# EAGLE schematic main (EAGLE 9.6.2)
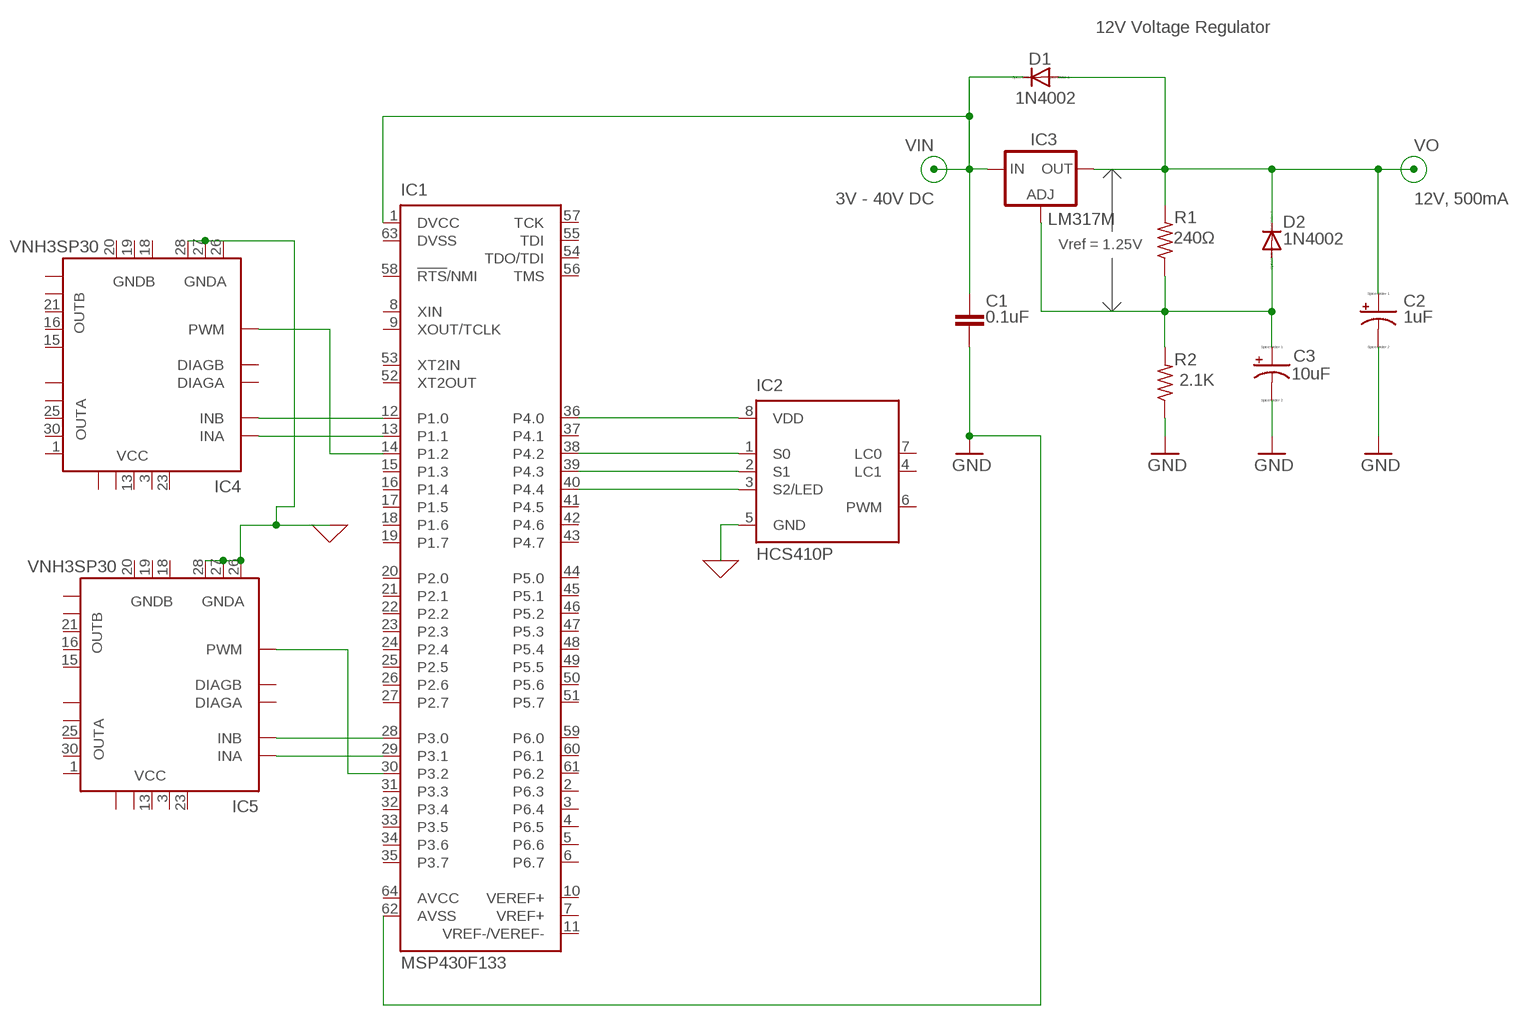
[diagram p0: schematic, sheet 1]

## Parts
C1  0.1uF  C-EU075-052X106  [C075-052X106]
C2  1uF  CPOL-US085CS-1AR  [085CS_1AR]
C3  10uF  CPOL-US085CS-1AR  [085CS_1AR]
D1  1N4002  1N4004  [DO41-10]
D2  1N4002  1N4004  [DO41-10]
IC1  MSP430F133  [SQFP-S-10X10-64]
IC2  HCS410P  [DIL8]
IC3  LM317MBSTT3  [SOT223]
IC4  VNH3SP30  [MULTIPOWERSO-30]
IC5  VNH3SP30  [MULTIPOWERSO-30]
R1  240Ω  R-US_M0805  [M0805]
R2  2.1K  R-US_M0805  [M0805]

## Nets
0: IC2.5(GND) IC4.26(GNDA) IC4.27(GNDA) IC4.28(GNDA) IC5.26(GNDA) IC5.27(GNDA) IC5.28(GNDA) ; supply symbol labelled GND
GND: C1.2 C2.- C3.- IC1.62(AVSS) R2.1
N$1: IC1.36(P4.0) IC2.8(VDD)
N$2: C3.+ D2.A IC3.1(ADJ) R1.1 R2.2
N$3: IC1.38(P4.2) IC2.1(S0)
N$4: IC1.39(P4.3) IC2.2(S1)
N$5: IC1.40(P4.4) IC2.3(S2/LED)
N$6: IC1.28(P3.0) IC5.11(INB)
N$7: IC1.29(P3.1) IC5.5(INA)
N$8: IC1.30(P3.2) IC5.8(PWM)
N$9: IC1.12(P1.0) IC4.11(INB)
N$10: IC1.13(P1.1) IC4.5(INA)
N$11: IC1.14(P1.2) IC4.8(PWM)
VIN: C1.1 D1.C IC1.1(DVCC) IC3.3(IN)
VO: C2.+ D1.A D2.C IC3.4(OUT) R1.2
Unconnected: IC1.2(P6.3) IC1.3(P6.4) IC1.4(P6.5) IC1.5(P6.6) IC1.6(P6.7) IC1.7(VREF+) IC1.8(XIN) IC1.9(XOUT/TCLK) IC1.10(VEREF+) IC1.11(VREF-/VEREF-) IC1.15(P1.3) IC1.16(P1.4) IC1.17(P1.5) IC1.18(P1.6) IC1.19(P1.7) IC1.20(P2.0) IC1.21(P2.1) IC1.22(P2.2) IC1.23(P2.3) IC1.24(P2.4) IC1.25(P2.5) IC1.26(P2.6) IC1.27(P2.7) IC1.31(P3.3) IC1.32(P3.4) IC1.33(P3.5) IC1.34(P3.6) IC1.35(P3.7) IC1.37(P4.1) IC1.41(P4.5) IC1.42(P4.6) IC1.43(P4.7) IC1.44(P5.0) IC1.45(P5.1) IC1.46(P5.2) IC1.47(P5.3) IC1.48(P5.4) IC1.49(P5.5) IC1.50(P5.6) IC1.51(P5.7) IC1.52(XT2OUT) IC1.53(XT2IN) IC1.54(TDO/TDI) IC1.55(TDI) IC1.56(TMS) IC1.57(TCK) IC1.58(!RTS!/NMI) IC1.59(P6.0) IC1.60(P6.1) IC1.61(P6.2) IC2.4(LC1) IC2.6(PWM) IC2.7(LC0) IC4.1(OUTA) IC4.6(DIAGA) IC4.10(DIAGB) IC4.15(OUTB) IC4.16(OUTB) IC4.21(OUTB) IC4.25(OUTA) IC4.30(OUTA) IC4.OUTA IC4.OUTA@1(OUTA) IC4.OUTB IC4.OUTB@1(OUTB) IC5.1(OUTA) IC5.6(DIAGA) IC5.10(DIAGB) IC5.15(OUTB) IC5.16(OUTB) IC5.21(OUTB) IC5.25(OUTA) IC5.30(OUTA) IC5.OUTA IC5.OUTA@1(OUTA) IC5.OUTB IC5.OUTB@1(OUTB)

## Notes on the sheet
- 12V Voltage Regulator
- 3V - 40V DC | 12V, 500mA
- Vref = 1.25V

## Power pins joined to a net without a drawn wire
AVCC: IC1.64(AVCC)
DVSS: IC1.63(DVSS)
GNDB: IC4.18(GNDB) IC4.19(GNDB) IC4.20(GNDB) IC5.18(GNDB) IC5.19(GNDB) IC5.20(GNDB)
VCC: IC4.3(VCC) IC4.13(VCC) IC4.23(VCC) IC4.VCC IC4.VCC@1(VCC) IC5.3(VCC) IC5.13(VCC) IC5.23(VCC) IC5.VCC IC5.VCC@1(VCC)

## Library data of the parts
C1 = rcl:C-EU: CAPACITOR, European symbol
C2 C3 = resistor:CPOL-US: POLARIZED CAPACITOR, American symbol
D1 D2 = diode:1N4004: DIODE
IC1 = texas:MSP430F1*: MIXED SIGNAL MICROCONTROLLER Family Members Include: - MSP430F133: 8KB+256B Flash Memory, 256B RAM - MSP430F135: 16KB+256B Flash Memory, 512B RAM - MSP430F147, MSP430F1471: 32KB+256B Flash Memory, 1KB RAM - MSP430F148, MSP430F1481: 48KB+256B Flash Memory, 2KB RAM - MSP430F149, MSP430F1491: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; MF: TEXAS INSTRUMENTS; MPN: MSP430F133IPM; OC_FARNELL: 1471268; OC_NEWARK: 75C4034
IC2 = microchip:HCS410: ENCODER code hopping encoder and transponder; MF: MICROCHIP; MPN: HCS410-I/P; OC_FARNELL: unknown; OC_NEWARK: 96K3679
IC3 = v-reg:LM317?*: 500 mA Adjustable Output Positive Voltage Regulator Source: http://www.onsemi.co.jp .. LM317M-D.PDF; PARTNUMBER: LM317M
IC4 IC5 = st-microelectronics:VNH3SP30: FULLY INTEGRATED H-BRIDGE MOTOR DRIVER Source: http://pdf1.alldatasheet.com/datasheet-pdf/view/84563/STMICROELECTRONICS/VNH3SP30.html; MPN: VNH3SP30-E; OC_FARNELL: 1739420; OC_NEWARK: 33R1486
R1 R2 = resistor:R-US_: RESISTOR, American symbol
